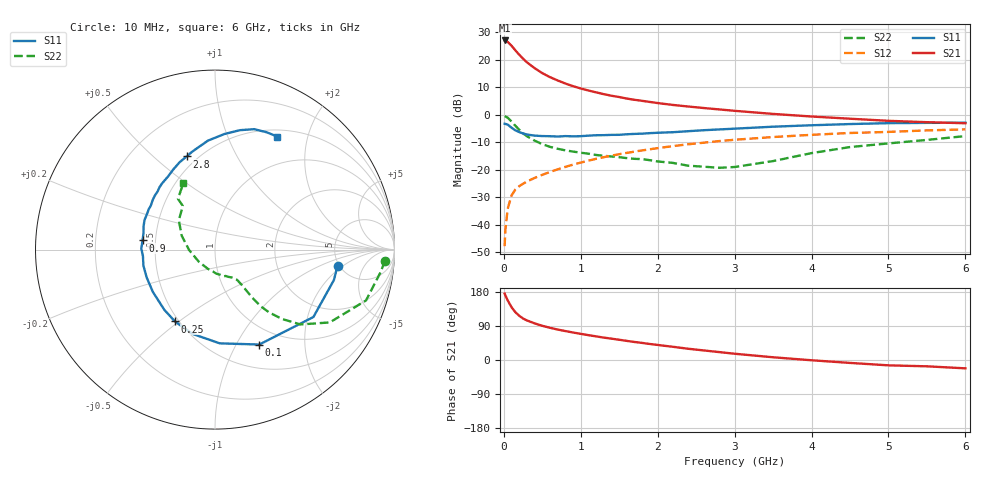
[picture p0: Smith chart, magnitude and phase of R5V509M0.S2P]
! SIEMENS Small Signal Semiconductors
! BFR183
! Si NPN RF Bipolar Junction Transistor in SOT23
! VCE = 0.5 V  IC = 9 mA
! Common Emitter S-Parameters:  May  1996
# GHz  S  MA  R  50
!  f  S11  S21  S12  S22
! GHz  MAG  ANG  MAG  ANG  MAG  ANG  MAG  ANG
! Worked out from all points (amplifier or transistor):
!   36 points, 10 MHz to 6 GHz, reference 50 ohm
!   highest |S21| = 27.0 dB at 10 MHz (marker M1)
!   |S21| within 3 dB of that: start of sweep to 132 MHz
!   unconditionally stable (mu >= 1): 624.2 MHz to 3.65 GHz
!   at 250 MHz: K = 0.64, MSG = 22.7 dB, |S12| = -25.1 dB
!   at 1.4 GHz: K = 1.11, MAG = 8.8 dB, |S12| = -14.8 dB
!   at 6 GHz: K = 0.99, MSG = 1.1 dB, |S12| = -5.3 dB
!   S11 on the Smith chart (normalised r, x): 10 MHz: 4.83, -1.65; 100 MHz: 0.78, -1.25; 250 MHz: 0.48, -0.48; 900 MHz: 0.42, +0.05; 2.8 GHz: 0.44, +0.64; 6 GHz: 0.59, +1.53
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0.01  0.6885 -7.5  22.48 175.4  0.0041 84.3  0.9486 -3.8
0.02  0.684 -14.3  22.14 170.4  0.0081 85.0  0.9315 -7.7
0.05  0.6646 -34.4  21.13 157.4  0.0196 74.3  0.8878 -18.6
0.1  0.5836 -65.0  18.06 139.3  0.0343 64.1  0.7573 -32.4
0.15  0.523 -87.1  14.82 126.0  0.0439 57.8  0.6331 -41.2
0.2  0.486 -105.0  12.4 116.7  0.0505 54.5  0.5372 -46.0
0.25  0.4584 -119.1  10.45 109.5  0.0559 53.5  0.4609 -49.3
0.3  0.4386 -130.0  9.012 104.4  0.0614 53.5  0.4082 -51.0
0.4  0.4189 -145.7  7.053 96.7  0.0713 54.7  0.3397 -52.2
0.5  0.4111 -157.8  5.719 90.2  0.0812 55.8  0.2929 -52.5
0.6  0.4088 -167.3  4.846 85.0  0.0916 57.0  0.2619 -52.7
0.7  0.4031 -174.9  4.212 80.3  0.1022 57.8  0.2417 -53.0
0.9  0.4068 172.8  3.32 72.5  0.1245 57.8  0.2147 -53.6
1.1  0.4185 162.0  2.768 65.6  0.1471 57.6  0.1965 -56.5
1.3  0.4273 153.1  2.375 59.1  0.1699 56.4  0.18 -59.4
1.6  0.4434 141.6  1.974 50.4  0.2036 53.9  0.1632 -66.3
2.2  0.4836 122.9  1.512 34.8  0.27 47.5  0.1336 -87.4
2.8  0.5426 106.9  1.254 20.9  0.3333 39.6  0.1089 -127.4
3.5  0.6084 93.7  1.039 7.2  0.395 29.6  0.1444 -179.1
4.5  0.6797 78.2  0.85 -7.7  0.468 16.1  0.2596 140.9
5.5  0.7142 66.3  0.735 -16.7  0.5215 5.0  0.3501 126.1
6  0.7193 61.1  0.703 -22.0  0.544 -2.4  0.4107 115.4
